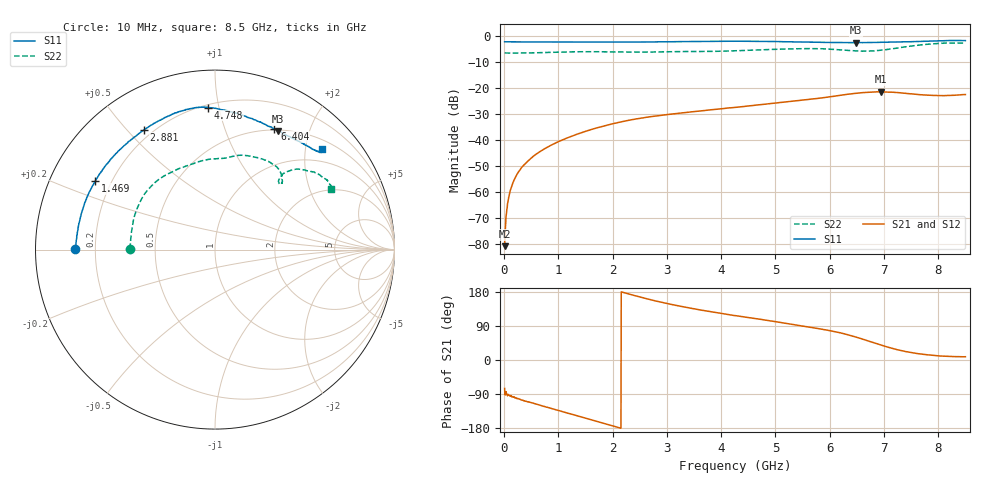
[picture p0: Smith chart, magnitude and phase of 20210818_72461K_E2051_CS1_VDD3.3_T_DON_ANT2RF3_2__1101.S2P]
!Agilent Technologies,E5071C,MY46417908,A.11.23
!Date: Wed Aug 18 14:30:41 2021
!Data & Calibration Information:
!Freq	S11:SOLT2(ON)	S21:SOLT2(ON)	S12:SOLT2(ON)	S22:SOLT2(ON)
!PortZ  Port1:50+j0  Port2:50+j0
!Above PortZ is port z conversion or system Z0 setting when saving the data.
!When reading, reference impedance value at option line is always used.
# Hz S dB R 50
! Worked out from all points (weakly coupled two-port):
!   1601 points, 10 MHz to 8.5 GHz, reference 50 ohm
!   highest |S21| = -21.41 dB at 6.94 GHz (marker M1); lowest = -80.7 dB at 10 MHz (marker M2)
!   lowest |S11| = -2.5 dB at 6.489 GHz (marker M3), VSWR 6.92, Z = 25.7 + j77 ohm
!   |S11| at or under -10 dB: nowhere
!   |S22| runs from -6.5 to -2.6 dB; largest |S21 - S12| = 0.00051
!   S11 on the Smith chart (normalised r, x): 10 MHz: 0.12, +0.00; 1.469 GHz: 0.14, +0.26; 2.881 GHz: 0.17, +0.56; 4.748 GHz: 0.22, +0.93; 6.404 GHz: 0.49, +1.49; 8.5 GHz: 0.69, +2.35
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1e7  -2.17 179.7  -80.71 -74.9  -80.40 -92.8  -6.47 179.6
7.3675e7  -2.21 178.4  -63.45 -90.8  -62.90 -91.7  -6.49 177.9
1.16125e8  -2.21 177.5  -59.20 -94.2  -59.41 -94.3  -6.50 176.7
2.01025e8  -2.23 175.8  -54.63 -99.7  -54.60 -99.0  -6.51 174.4
3.124562e8  -2.25 173.4  -50.80 -105.3  -50.80 -105.0  -6.50 171.6
5.300125e8  -2.24 169.1  -46.33 -113.5  -46.33 -113.5  -6.43 166.1
7.369562e8  -2.26 164.7  -43.42 -122.6  -43.41 -122.2  -6.32 160.1
1.426769e9  -2.28 151.0  -37.11 -150.4  -37.12 -150.4  -6.01 138.7
1.469219e9  -2.29 150.1  -36.82 -152.1  -36.81 -152.2  -6.01 137.4
2.185562e9  -2.29 135.2  -32.82 178.7  -32.83 178.6  -6.13 116.3
2.843538e9  -2.22 121.3  -30.57 154.2  -30.58 154.1  -6.07 101.5
2.880681e9  -2.21 120.6  -30.51 153.0  -30.50 153.0  -6.06 100.9
4.255e9  -1.97 98.6  -27.39 117.2  -27.39 117.1  -5.63 80.7
4.748481e9  -2.02 92.8  -26.27 106.9  -26.27 106.9  -5.23 73.6
5.671769e9  -2.33 78.7  -24.21 85.7  -24.23 85.7  -4.81 54.9
6.404031e9  -2.50 63.8  -22.16 63.8  -22.18 63.6  -5.58 44.8
6.488931e9  -2.53 62.0  -21.99 60.2  -22.01 60.1  -5.71 44.8
6.939962e9  -2.38 53.3  -21.41 39.6  -21.43 39.4  -5.45 47.7
7.088538e9  -2.31 51.1  -21.50 33.3  -21.51 33.1  -5.05 48.1
7.592631e9  -2.09 44.7  -22.37 17.4  -22.37 17.3  -3.59 42.3
8.0755e9  -1.78 42.2  -22.89 10.3  -22.87 10.2  -2.75 32.9
8.5e9  -1.74 43.2  -22.46 8.6  -22.43 8.3  -2.76 27.6
